|   National Semiconductor Corporation
|   Networks Products Group
|   IBIS Model for MacPhyter DP83815DVNG
|   144 TQFP Package
| IBIS file dp83815d.ibs was created using s2ibis2 version 2.1
| North Carolina State University Electronics Research Laboratory 1997
| http://www.eigroup.org/ibis/tools.htm -> SPICE-toIBISconversion(IBISv2.1)
| s2ibis2.tar.Z   11FEB97   652K
| s2ibis2_fix.tar.Z 13MAY97   119K
[IBIS ver]   2.1
[File_name]   dp83815v.ibs
[File Rev]   1.0
[Date]   March 15, 2001
[Source]   Originated at National Semiconductor
[Notes]   For questions or comments contact
   Alan.E.Segervall@nsc.com or phone 408-721-7082
   Spectre s2ibis simulations, created by Alan E Segervall.
[Disclaimer]  Absolutely no guarantees, for modeling purposes only.
   National Semiconductor Corporation hereby grants the user of this IBIS
model a non-exclusive, nontransferable license to use this IBIS model under
the following terms. Before using this IBIS model, the user should read this
license.  If the user does not accept these terms,  the IBIS model should be
returned to National within 30 days.
   The user is granted this license only to use the IBIS model and is not
granted rights to sell, load, rent, lease or license the IBIS model in whole
or in part, or in modified form to anyone other than user. User may modify
the IBIS model to suit its specific applications but rights to derivative
works and such modifications shall belong to National.
   This IBIS model is provided on an "AS IS" basis and National makes
absolutely no warranty with respect to the information contained herein.
NATIONAL DISCLAIMS AND CUSTOMER WAIVES ALL WARRANTIES, EXPRESS OR IMPLIED,
INCLUDING WARRANTIES OF MERCHANTABILITY OR FITNESS FOR A PARTICULAR PURPOSE.
The entire risk as to quality and performance is with the Customer.
ACCORDINGLY, IN NO EVENT SHALL THE COMPANY BE LIABLE FOR ANY DAMAGES, WHETHER
IN CONTRACT OR COURT, INCLUDING ANY LOST PROFITS OR OTHER INCIDENTAL,
CONSEQUENTIAL, EXEMPLARY, OR PUNITIVE DAMAGES ARISING OUT OF THE USE OR
APPLICATION OF THE IBIS model provided in this package. Further, National
reserves the right to make changes without notice to any product herein to
improve reliability, function, or design. National does not convey any license
under patent rights or any other intellectual property rights, including those
of third parties.
   National is not obligated to provide maintenance or support
for the licensed IBIS model.
[Copyright]   Copyright 2001, National Semiconductor Corporation, All rights
   reserved
|   Component DP83815DVNG
[Component] DP83815DVNG
[Manufacturer] National Semiconductor Corp.
[Package]
| variable   typ   min   max
R_pkg   0.0186  0.0165  0.0212
L_pkg   5.1673n 4.5845n 5.8930n
C_pkg   1.4668p 1.1660p 1.6850p
[Pin]   signal_name   model_name   R_pin   L_pin   C_pin
1	MA3/EDDI   XWBHOV8   0.09417	10.56856n   1.45734p
2   MA4/EECLK   XWBHOV8   0.09174	11.20123n   1.97801p
3   MA5   XWBBOV125   0.08958	10.97567n   1.94215p
4   MDIO   XWBHOV12   0.08741	10.71967n   1.90048p
5   MDC   XWBHOV12   0.08552	10.51450n   1.87149p
6   RXCLK   XWBHOV12   0.08394	10.35103n   1.84693p
7   RXD0/MA6   XWBHOV12   0.08249	10.16823n   1.81372p
8   VSSIO1   GND   0.08092   9.99595n   1.77943p
9   VDDIO1   POWER   0.07970   9.83102n   1.73813p
10   RXD1/MA7   XWBHOV12   0.07863   9.67184n   1.70854p
11   RXD2/MA8   XWBHOV12   0.07780   9.54668n   1.68294p
12   RXD3/MA9   XWBHOV12   0.07705   9.43396n   1.65931p
13   RXOE   XWBHOV12   0.07650   9.34133n   1.63780p
14   RXER/MA10   XWBHOV12   0.07609   9.25849n   1.61819p
15   RXDV/MA11   XWBHOV12   0.07576   9.18982n   1.60194p
16   VSSIO2   GND   0.07563   9.14528n   1.58960p
17   X1   OSC25_XI   0.07564   9.11890n   1.57901p
18   X2   OSC25_XO   0.07571   9.05959n   1.54800p
19   VDDIO2   POWER   0.07569   9.05220n   1.54735p
20   PHYVSS1   GND   0.07557   9.11070n   1.57844p
21   PHYVDD1   POWER   0.07552   9.13490n   1.58896p
22   TXD0/MA12   XWBHOV12   0.07560   9.17754n   1.60128p
23   TXD1/MA13   XWBHOV12   0.07588   9.24547n   1.61760p
24   TXD2/MA14   XWBHOV12   0.07625   9.32613n   1.63715p
25   TXD3/MA15   XWBHOV12   0.07676   9.41837n   1.65876p
26   VSSIO3   GND   0.07746   9.53130n   1.68255p
27   VDDIO3   POWER   0.07825   9.65482n   1.70812p
28   COL/MA16   XWBHOV12   0.07927   9.81446n   1.73789p
29   CRS   XWBHOV12   0.08045   9.97971n   1.77936p
30   TXEN   XWBHOV12   0.08198	10.15047n   1.81363p
31   TXCLK   XWBHOV12   0.08342	10.33543n   1.84708p
32   PHYVSS2   GND   0.08496	10.50193n   1.87205p
33   PHYVDD2   POWER   0.08681   9.28202n   1.76578p
34	NC   NC   0.09006   11.00835n   1.94375p
35   FXVSS   GND   0.09259	11.30637n   1.98533p
36   FXVDD   POWER   0.09397	10.56623n   1.45773p
37   SUBGND1   GND   0.09234	10.45740n   1.45250p
38   RXAVSS1   GND   0.09118	11.18123n   1.97786p
39   RXAVDD1   POWER   0.09006	11.00835n   1.94375p
40   VREF   CORESIG   0.08772	10.74355n   1.90179p
41   RESERVED   NC   0.08514   10.58185n   1.89448p
42   NC   NC   0.08318   10.36692n   1.86481p
43   NC   NC   0.08153   10.19237n   1.83940p
44   RXAVSS2   GND   0.07814   9.80329n   1.76981p
45   TPRDM   RD   0.07772   9.68048n   1.72999p
46   TPRDP   RD   0.07658   9.51591n   1.70012p
47   RXAVDD2   POWER   0.07569   8.15856n   1.55767p
48   NC   NC   0.07439   9.23933n   1.64916p
49   SUBGND2   GND   0.07356   9.12297n   1.62625p
50   NC   NC   0.07347   9.06263n   1.60779p
51   TXDVSS   GND   0.07329   9.00316n   1.59193p
52   TXIOVSS1   GND   0.07316   8.95820n   1.57957p
53   TPTDM   SIGOVSB   0.07316   8.93182n   1.56897p
54   TPTDP   SIGOVSB   0.07325   8.87366n   1.53802p
55   TXIOVSS2   GND   0.07323   8.86597n   1.53736p
56   TXDVDD   POWER   0.07310   8.92471n   1.56847p
57   MACVSS1   GND   0.07307   8.94999n   1.57907p
58   MACVDD1   POWER   0.07317   8.99385n   1.59143p
59   PMEN/CLKRUNN  XWPME   0.07347   9.06263n   1.60779p
60   PCICLK   XWPCICLK   0.07384   9.14413n   1.62738p
61   INTAN   XWPCIIO   0.07439   9.23933n   1.64916p
62   RSTN   XWBHOV2   0.07514   9.35608n   1.67315p
63   GNTN   XWPCIIO   0.07598   9.48383n   1.69895p
64   REQN   XWPCIIO   0.07711   9.65108n   1.72912p
65   PCIVSS1   GND   0.07837   9.82226n   1.77091p
66   AD31   XWPCIIO   0.07999   9.99980n   1.80555p
67   AD30   XWPCIIO   0.08153	10.19237n   1.83940p
68   AD29   XWPCIIO   0.08318	10.36692n   1.86481p
69   PCIVDD1   POWER   0.08514	10.58185n   1.89448p
70   AD28   XWPCIIO   0.08740	10.84756n   1.93681p
71   AD27   XWPCIIO   0.08964	11.08374n   1.97339p
72   AD26   XWPCIIO   0.09222	10.46879n   1.45395p
73   AD25   XWPCIIO   0.09371	10.53391n   1.45550p
74   AD24   XWPCIIO   0.09129	11.16816n   1.97625p
75   CBEN3   XWPCIIO   0.08916	10.94410n   1.94049p
76   IDSEL   XWPCIIO   0.08701	10.69010n   1.89891p
77   PCSVSS2   GND   0.08515	10.48674n   1.87003p
78   AD23   XWPCIIO   0.08360	10.32467n   1.84551p
79   AD22   XWPCIIO   0.08214	10.14216n   1.81235p
80   PCIVDD2   POWER   0.08059   9.97260n   1.77823p
81   AD21   XWPCIIO   0.07943   9.81119n   1.73709p
82   AD20   XWPCIIO   0.07838   9.65382n   1.70760p
83   AD19   XWPCIIO   0.07758   9.53077n   1.68212p
84   VSSIO4   GND   0.07686   9.42017n   1.65860p
85   VDDIO4   POWER   0.07634   9.32966n   1.63720p
86   AD18   XWPCIIO   0.07596   9.24893n   1.61770p
87   AD17   XWPCIIO   0.07565   9.18178n   1.60151p
88   AD16   XWPCIIO   0.07556   9.13978n   1.58930p
89   CBEN2   XWPCIIO   0.07559   9.11551n   1.57883p
90   PCIVSS3   GND   0.07570   9.05952n   1.54801p
91   FRAMEN   XWPCIIO   0.07570   9.05328n   1.54741p
92   IRDYN   XWPCIIO   0.07559   9.11287n   1.57858p
93   TRDYN   XWPCIIO   0.07557   9.13876n   1.58919p
94   PCIVDD3   POWER   0.07566   9.18262n   1.60155p
95   DEVSELN   XWPCIIO   0.07597   9.25182n   1.61794p
96   STOPN   XWPCIIO   0.07635   9.33375n   1.63755p
97   PERRN   XWPCIIO   0.07688   9.42768n   1.65926p
98   SERRN   XWPCIIO   0.07760   9.54188n   1.68312p
99   PAR   XWPCIIO   0.07838   9.66498n   1.70866p
100   CBEN1   XWPCIIO   0.07943   9.82631n   1.73852p
101   AD15   XWPCIIO   0.08062   9.99283n   1.78006p
102   AD14   XWPCIIO   0.08217	10.16444n   1.81438p
103   PCIVSS4   GND   0.08362	10.35067n   1.84789p
104   AD13   XWPCIIO   0.08518	10.51844n   1.87293p
105   AD12   XWPCIIO   0.08705	10.72576n   1.90220p
106   AD11   XWPCIIO   0.08919	10.98300n   1.94408p
107   PCIVDD4   POWER   0.09133	11.21114n   1.98023p
108   AD10   XWPCIIO   0.09375	10.55211n   1.45711p
109   AD9   XWPCIIO   0.09226	10.42111n   1.44930p
110   AD8   XWPCIIO   0.08968	11.04698n   1.96978p
111   CBEN0   XWPCIIO   0.08758	10.82151n   1.93378p
112   AD7   XWPCIIO   0.08528	10.55631n   1.89162p
113   AD6   XWPCIIO   0.08328	10.34369n   1.86228p
114   PCIVSS5   GND   0.08165	10.17606n   1.83749p
115   AD5   XWPCIIO   0.08013   9.98770n   1.80396p
116   AD4   XWPCIIO   0.07847   9.81008n   1.76944p
117   PCIVDD5   POWER   0.07722   9.64395n   1.72810p
118   AD3   XWPCIIO   0.07615   9.48356n   1.69840p
119   AD2   XWPCIIO   0.07527   9.35453n   1.67260p
120   AD1   XWPCIIO   0.07448   9.23909n   1.64883p
121   AD0   XWPCIIO   0.07390   9.14579n   1.62735p
122   3VAUX   XWBHOV4   0.07353   9.06494n   1.60780p
123   PWRGOOD   XWBHOV4   0.07320   8.99597n   1.59154p
124   MACVSS2   GND   0.07308   8.95228n   1.57925p
125   MACVDD2   POWER   0.07310   8.92759n   1.56875p
126   SUBGND3   GND   0.07312   8.86440n   1.53754p
127   RESERVED   NC   0.07310   8.92759n   1.56875p
128   EESEL   XWBHOV8   0.07307   8.92157n   1.56828p
129   MCSN   XWBHOV8   0.07301   8.94474n   1.57876p
130   MRDN   XWBHOV8   0.07308   8.98708n   1.59107p
131   MWRN   XWBHOV8   0.07338   9.05628n   1.60745p
132   MD0   XWBHOV8   0.07377   9.13905n   1.62711p
133   MD1/CFGDISN   XWBHOV8   0.07433   9.23468n   1.64891p
134   MD2   XWBHOV8   0.07509   9.35227n   1.67295p
135   MD3   XWBHOV8   0.07594   9.48086n   1.69879p
136   VSSIO5   GND   0.07706   9.64727n   1.72892p
137   VDDIO5   POWER   0.07834   9.82057n   1.77082p
138   MD4/EEDO   XWBHOV8   0.07999   9.99980n   1.80555p
139   MD5   XWBHOV8   0.08156	10.19449n   1.83952p
140   MD6   XWBHOV8   0.08324	10.37199n   1.86508p
141   MD7   XWBHOV8   0.08521	10.58693n   1.89475p
142   MA0/LEDACTN   XWBHOV8   0.08751	10.85560n   1.93724p
143   MA1/LED10N   XWBHOV8   0.08980	11.09559n   1.97403p
144   MA2/LED100N   XWBHOV8   0.09238	10.48064n   1.45459p
| Models and submodels in the file (13): XWBHOV2 (I/O), XWBHOV4 (I/O), XWBHOV8 (I/O), XWBHOV12 (I/O), XWBBOV125 (I/O), XWPCIIO (I/O), XWPME (I/O_open_drain), XWPCICLK (Input), RD (Input), CORESIG (Input), SIGOVSB (Input), OSC25_XO (Output), OSC25_XI (Input)
